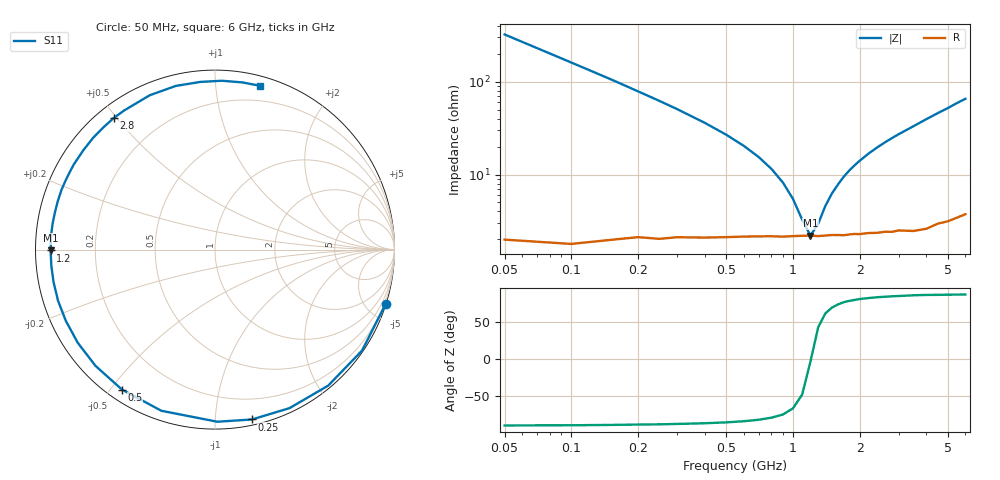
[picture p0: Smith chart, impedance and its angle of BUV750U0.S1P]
! Infineon Technologies  Discrete & RF Semiconductors
! BB 833
! Si Tuning Diode in SOD323
! VR = 0.75 V
! S-Parameters:  June  1999
# GHz  S  MA  R  50
!  f  S11
! GHz  MAG  ANG
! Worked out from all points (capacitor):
!   34 points, 50 MHz to 6 GHz, reference 50 ohm
!   read as one part to ground: C = 9.82 pF near 50 MHz
!   lowest |Z| = 2.2 ohm at 1.2 GHz (marker M1)
!   series resonance near 1.206 GHz, so ESL is about 1.8 nH
!   S11 on the Smith chart (normalised r, x): 50 MHz: 0.04, -6.46; 250 MHz: 0.04, -1.24; 500 MHz: 0.04, -0.54; 1.2 GHz: 0.04, -0.00; 2.8 GHz: 0.05, +0.49; 6 GHz: 0.07, +1.31
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0.05  0.9981 -17.6
0.1  0.9937 -34.5
0.15  0.9859 -50.2
0.2  0.976 -64.8
0.25  0.9686 -77.7
0.3  0.9592 -89.2
0.4  0.9464 -108.4
0.5  0.9363 -123.6
0.6  0.9289 -135.8
0.7  0.9242 -145.9
0.8  0.9209 -154.5
0.9  0.9198 -161.9
1  0.9176 -168.5
1.2  0.9158 -179.7
1.4  0.9162 170.8
1.6  0.9164 162.8
1.8  0.9171 155.4
2  0.9188 148.9
2.2  0.9191 142.9
2.4  0.9215 137.4
2.8  0.9252 127.5
3  0.9256 123.0
3.5  0.9337 112.9
4  0.9378 103.4
4.5  0.9377 95.0
5  0.9415 87.7
5.5  0.9441 80.6
6  0.9464 74.7
